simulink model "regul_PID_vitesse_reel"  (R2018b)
settings: Solver=ode5  StartTime=0.0  StopTime=inf  FixedStep=0.005  RelTol=1e-3  AbsTol=1e-6
undefined symbols (not defined in the file or in its folder): RTDAC4PCIBaseAddress
libraries: simulink x1

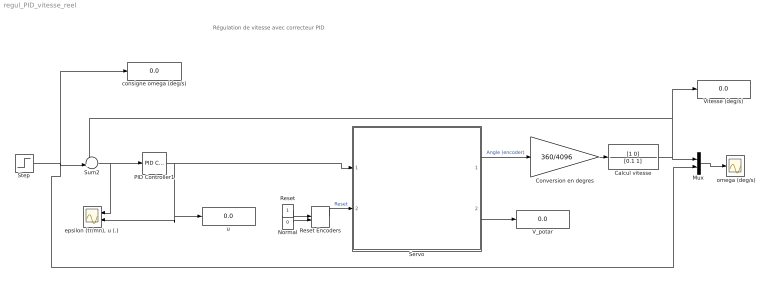
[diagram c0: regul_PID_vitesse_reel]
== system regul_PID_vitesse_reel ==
  note: Régulation de vitesse avec correcteur PID
  " omega (deg/s)" : Scope
  Calcul vitesse : TransferFcn  Numerator=[1 0]  Denominator=[0.1 1]
  Conversion en degres : Gain  Gain=360/4096
  Mux : Mux  Inputs=2
  Normal : Constant  Value=0
  PID Controller1 : simulink/Continuous/PID Controller  Controller=PID  Form=Parallel  TimeDomain=Continuous-time  SampleTime=-1  IntegratorMethod=Forward Euler  FilterMethod=Forward Euler  ControllerParametersSource=internal  P=1  I=1  D=0  UseFilter=on  N=100  TunerSelectOption=Transfer Function Based (PID Tuner App)  InitialConditionSource=internal  InitialConditionForIntegrator=0  InitialConditionForFilter=0  DifferentiatorICPrevScaledInput=0  ExternalReset=none  TrackingMode=off  Kt=1  LimitOutput=off  UpperSaturationLimit=inf  LowerSaturationLimit=-inf  LinearizeAsGain=on  AntiWindupMode=none  Kb=1  POutMin=[]  POutMax=[]  IOutMin=[]  IOutMax=[]  DOutMin=[]  DOutMax=[]  NOutMin=[]  NOutMax=[]  SumOutMin=[]  SumOutMax=[]  SaturationOutMin=[]  SaturationOutMax=[]  PParamMin=[]  PParamMax=[]  IParamMin=[]  IParamMax=[]  DParamMin=[]  DParamMax=[]  NParamMin=[]  NParamMax=[]  KbParamMin=[]  KbParamMax=[]  KtParamMin=[]  KtParamMax=[]  KbOutMin=[]  KbOutMax=[]  KtOutMin=[]  KtOutMax=[]  IntegratorOutMin=[]  IntegratorOutMax=[]  FilterOutMin=[]  FilterOutMax=[]  SumI1OutMin=[]  SumI1OutMax=[]  SumI2OutMin=[]  SumI2OutMax=[]  SumI3OutMin=[]  SumI3OutMax=[]  SumI4OutMin=[]  SumI4OutMax=[]  SumDOutMin=[]  SumDOutMax=[]  DifferentiatorOutMin=[]  DifferentiatorOutMax=[]  FilterDiffOutCoefMin=[]  FilterDiffOutCoefMax=[]  ReciprocalOutMin=[]  ReciprocalOutMax=[]  SumDenOutMin=[]  SumDenOutMax=[]  SumNumOutMin=[]  SumNumOutMax=[]  DivideOutMin=[]  DivideOutMax=[]  IntegratorContinuousStateAttributes=''  IntegratorStateMustResolveToSignalObject=off  IntegratorRTWStateStorageClass=Auto  FilterContinuousStateAttributes=''  FilterStateMustResolveToSignalObject=off  FilterRTWStateStorageClass=Auto  ParallelPVariant=InternalParameters  IdealPVariant=Disabled  IVariant=InternalParameters  DVariant=InternalParameters  IntegratorVariant=Continuous  SatVariant=Disabled  AWVariant=Passthrough  PCopyVariant=Disabled  TRVariant=Disabled  FdbkBlocksVariant=Forward  IdealPFdbkVariant=Disabled  SatFdbkVariant=Disabled  DerivativeFilterVariant=ContFilter  NVariant=InternalParameters  NCopyVariant=Disabled  FilterICVariant=InternalICsFilter  IntegratorICVariant=InternalICs  ExternalResetVariant=Disabled  TRSumVariant=Passthrough  SumFdbkVariant=Disabled  SumVariant=Sum_PID
  Reset : Constant
  Reset Encoders : ManualSwitch  CurrentSetting=0
  Servo : Subsystem  mask{BaseAddress=RTDAC4PCIBaseAddress(-1,-1), T0=0.005}
      mask prompts: BaseAddress "Base Address:"; T0 "Sampling Period:"
  Step : Step  Time=10  After=9000  SampleTime=0
  Sum2 : Sum  Inputs=-+|
  V_potar : Display
  Vitesse (deg/s) : Display
  consigne omega (deg/s) : Display
  "epsilon (tr/mn), u (.)" : Scope  NumInputPorts=2
  u : Display
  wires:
  Reset Encoders/1 -> Servo/2(Reset Encoder)  "Reset"
  Normal/1 -> Reset Encoders/2
  Reset/1 -> Reset Encoders/1
  Servo/1(Codeur_angulaire) -> Conversion en degres/1  "Angle (encoder)"
  Servo/2(Set-up) -> V_potar/1
  Conversion en degres/1 -> Calcul vitesse/1
  PID Controller1/1 -> Servo/1(PWM Control), u/1, "epsilon (tr/mn), u (.)"/2
  Sum2/1 -> PID Controller1/1, "epsilon (tr/mn), u (.)"/1
  Mux/1 -> " omega (deg/s)"/1
  Step/1 -> consigne omega (deg/s)/1, Mux/2, Sum2/2
  Calcul vitesse/1 -> Sum2/1, Vitesse (deg/s)/1, Mux/1

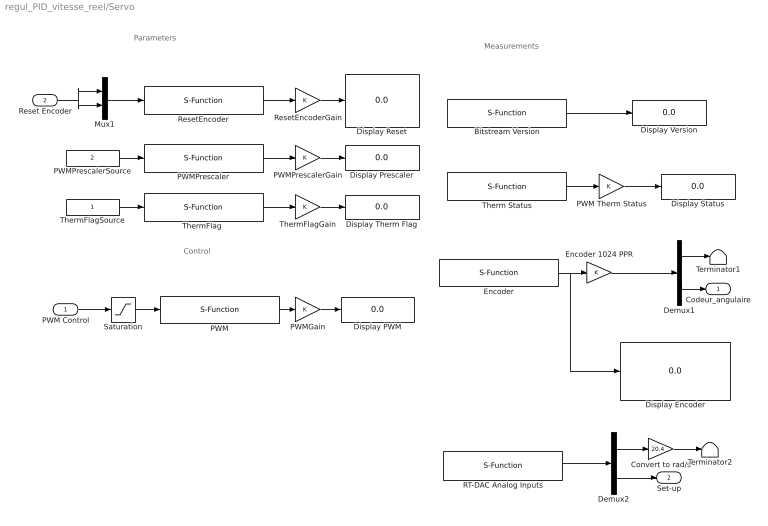
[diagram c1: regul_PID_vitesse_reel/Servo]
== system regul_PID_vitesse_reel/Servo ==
  note: Parameters
  note: Control
  note: Measurements
  PWM Control : Inport
  Reset Encoder : Inport  Port=2
  Bitstream Version : S-Function  FunctionName=Servo_BitstreamVersion  Parameters=BaseAddress, T0  SFunctionDeploymentMode=off  EnableBusSupport=off
  Convert to rad/s : Gain  Gain=20.4
  Demux1 : Demux  Outputs=2
  Demux2 : Demux  Outputs=2
  Display Encoder : Display
  Display PWM : Display
  Display Prescaler : Display
  Display Reset : Display
  Display Status : Display
  Display Therm Flag : Display
  Display Version : Display
  Encoder : S-Function  FunctionName=Servo_Encoder  Parameters=BaseAddress, T0  SFunctionDeploymentMode=off  EnableBusSupport=off
  Encoder 1024 PPR : Gain
  Mux1 : Mux  Inputs=2
  PWM : S-Function  FunctionName=Servo_PWM  Parameters=BaseAddress, T0  SFunctionDeploymentMode=off  EnableBusSupport=off
  PWM Therm Status : Gain
  PWMGain : Gain
  PWMPrescaler : S-Function  FunctionName=Servo_PWMPrescaler  Parameters=BaseAddress, T0  SFunctionDeploymentMode=off  EnableBusSupport=off
  PWMPrescalerGain : Gain
  PWMPrescalerSource : Constant  Value=2
  RT-DAC Analog Inputs : S-Function  FunctionName=servo_analoginputs  Parameters=BaseAddress, [1 0], [1 1], T0  SFunctionDeploymentMode=off  EnableBusSupport=off
  ResetEncoder : S-Function  FunctionName=Servo_ResetEncoder  Parameters=BaseAddress, T0  SFunctionDeploymentMode=off  EnableBusSupport=off
  ResetEncoderGain : Gain
  Saturation : Saturate  UpperLimit=1  LowerLimit=-1
  Terminator1 : Terminator
  Terminator2 : Terminator
  Therm Status : S-Function  FunctionName=Servo_PWMTherm  Parameters=BaseAddress, T0  SFunctionDeploymentMode=off  EnableBusSupport=off
  "ThermFlag " : S-Function  FunctionName=Servo_ThermFlag  Parameters=BaseAddress, T0  SFunctionDeploymentMode=off  EnableBusSupport=off
  ThermFlagGain : Gain
  ThermFlagSource : Constant
  Codeur_angulaire : Outport
  Set-up : Outport  Port=2
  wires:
  Encoder/1 -> Encoder 1024 PPR/1, Display Encoder/1
  Saturation/1 -> PWM/1
  PWM/1 -> PWMGain/1
  PWMGain/1 -> Display PWM/1
  ResetEncoder/1 -> ResetEncoderGain/1
  PWMPrescaler/1 -> PWMPrescalerGain/1
  Mux1/1 -> ResetEncoder/1
  PWMPrescalerSource/1 -> PWMPrescaler/1
  ResetEncoderGain/1 -> Display Reset/1
  PWMPrescalerGain/1 -> Display Prescaler/1
  PWM Control/1 -> Saturation/1
  Encoder 1024 PPR/1 -> Demux1/1
  Therm Status/1 -> PWM Therm Status/1
  PWM Therm Status/1 -> Display Status/1
  Bitstream Version/1 -> Display Version/1
  Reset Encoder/1 -> Mux1/1, Mux1/2
  "ThermFlag "/1 -> ThermFlagGain/1
  ThermFlagSource/1 -> "ThermFlag "/1
  ThermFlagGain/1 -> Display Therm Flag/1
  Demux1/1 -> Terminator1/1
  Demux1/2 -> Codeur_angulaire/1
  RT-DAC Analog Inputs/1 -> Demux2/1
  Demux2/2 -> Set-up/1
  Demux2/1 -> Convert to rad/s/1
  Convert to rad/s/1 -> Terminator2/1
